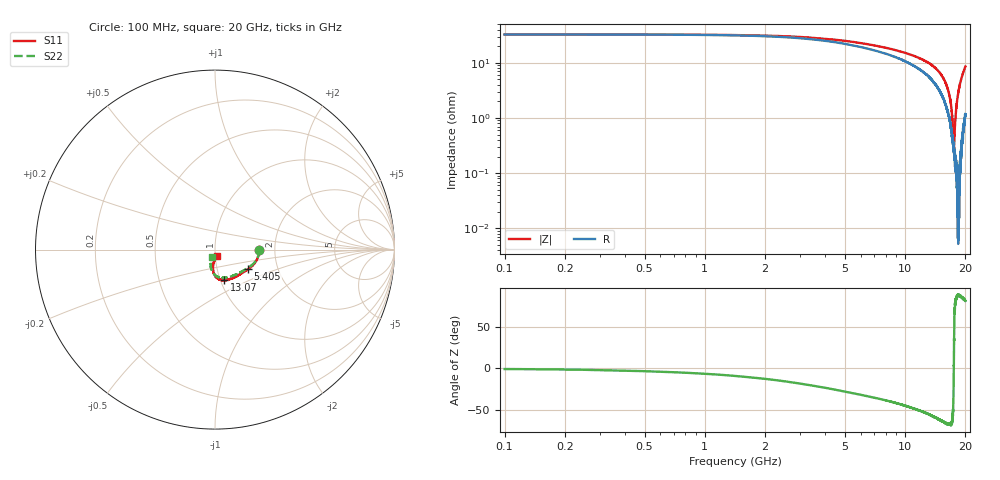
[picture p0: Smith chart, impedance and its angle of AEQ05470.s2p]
!Keysight Technologies,N5225A,MY51451420,A.10.40.12
!Date: Monday, February 01, 2016 13:10:57
!Correction: S11(Full 2 Port(1,2))
!S21(Full 2 Port(1,2))
!S12(Full 2 Port(1,2))
!S22(Full 2 Port(1,2))
!S2P File: Measurements: S11, S21, S12, S22:
# Hz S  dB  R 50
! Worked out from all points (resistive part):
!   3201 points, 100 MHz to 20 GHz, reference 50 ohm
!   read as one part in series: R = 32.7 ohm at 199.5 MHz
!   S11 on the Smith chart (normalised r, x): 100 MHz: 1.65, -0.01; 5.405 GHz: 1.41, -0.32; 13.07 GHz: 1.04, -0.37; 20 GHz: 1.02, -0.07
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1e8  -12.19 -0.5  -2.46 0.2  -2.45 0.2  -12.15 -0.5
1.853688e9  -12.30 -10.5  -2.31 2.4  -2.32 2.5  -12.30 -9.7
3.420812e9  -12.69 -19.9  -2.05 3.7  -2.05 3.7  -12.72 -18.4
5.404594e9  -13.39 -31.0  -1.68 4.0  -1.67 4.0  -13.51 -28.8
6.735406e9  -13.84 -38.3  -1.43 3.6  -1.43 3.6  -14.04 -35.5
7.848562e9  -14.14 -44.3  -1.24 3.1  -1.25 3.0  -14.40 -41.3
1.005e10  -14.52 -56.9  -0.93 1.6  -0.93 1.6  -14.96 -53.3
1.306609e10  -14.95 -73.2  -0.57 -1.1  -0.57 -1.1  -15.53 -70.2
1.337081e10  -15.04 -75.0  -0.53 -1.3  -0.54 -1.4  -15.63 -72.1
1.4428e10  -15.42 -80.4  -0.42 -2.4  -0.43 -2.5  -15.90 -78.4
1.520534e10  -15.80 -84.4  -0.33 -3.4  -0.33 -3.4  -16.25 -83.2
1.579612e10  -16.24 -87.4  -0.27 -4.2  -0.27 -4.2  -16.59 -87.1
1.668541e10  -17.18 -91.6  -0.18 -5.4  -0.18 -5.4  -17.36 -92.6
1.704609e10  -17.65 -93.3  -0.14 -6.0  -0.14 -6.0  -17.75 -95.0
1.755603e10  -18.62 -95.2  -0.10 -6.9  -0.10 -7.0  -18.50 -98.4
1.815303e10  -20.00 -96.2  -0.08 -8.1  -0.08 -8.1  -19.59 -102.4
1.85075e10  -21.02 -96.8  -0.08 -8.9  -0.07 -8.9  -20.46 -104.7
1.901122e10  -22.92 -95.2  -0.08 -9.9  -0.08 -9.9  -22.10 -107.8
1.939678e10  -24.79 -91.1  -0.10 -10.8  -0.09 -10.8  -23.59 -108.6
1.963931e10  -26.11 -87.1  -0.12 -11.3  -0.12 -11.3  -24.81 -109.6
1.991916e10  -27.81 -76.4  -0.16 -11.9  -0.15 -11.9  -26.57 -109.5
2e10  -28.36 -73.4  -0.16 -12.1  -0.16 -12.1  -27.13 -109.1
